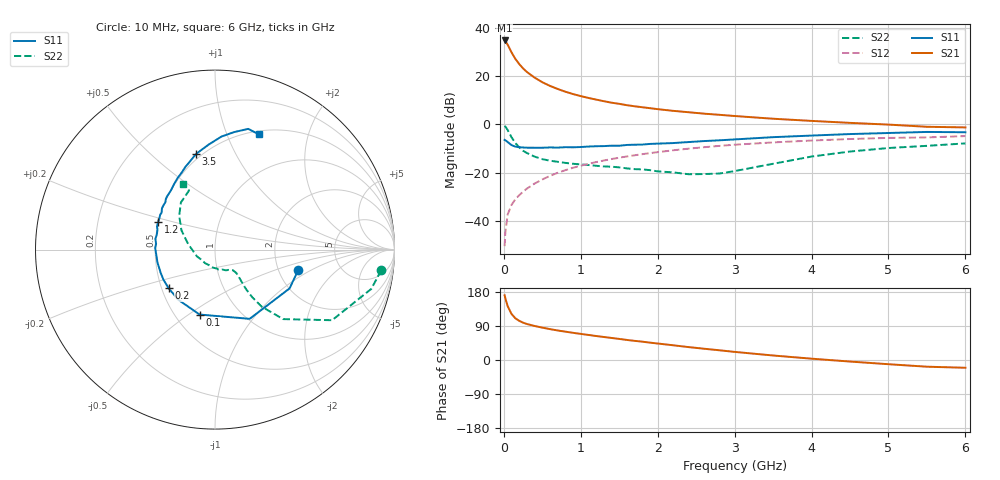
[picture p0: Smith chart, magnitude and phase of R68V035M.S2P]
! SIEMENS Small Signal Semiconductors
! BFR193
! Si NPN RF Bipolar Junction Transistor in SOT23
! VCE = 8 V  IC = 35 mA
! Common Emitter S-Parameters:  May  1996
# GHz  S  MA  R  50
!  f  S11  S21  S12  S22
! GHz  MAG  ANG  MAG  ANG  MAG  ANG  MAG  ANG
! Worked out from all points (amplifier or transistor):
!   36 points, 10 MHz to 6 GHz, reference 50 ohm
!   highest |S21| = 34.8 dB at 10 MHz (marker M1)
!   |S21| within 3 dB of that: start of sweep to 69.24 MHz
!   unconditionally stable (mu >= 1): 471.7 MHz to 2.129 GHz
!   at 250 MHz: K = 0.90, MSG = 25.5 dB, |S12| = -27.9 dB
!   at 1.4 GHz: K = 1.02, MAG = 10.8 dB, |S12| = -14.4 dB
!   at 6 GHz: K = 0.95, MSG = 1.8 dB, |S12| = -4.8 dB
!   S11 on the Smith chart (normalised r, x): 10 MHz: 2.56, -0.77; 100 MHz: 0.66, -0.55; 200 MHz: 0.54, -0.27; 1.2 GHz: 0.50, +0.18; 3.5 GHz: 0.47, +0.71; 6 GHz: 0.54, +1.30
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0.01  0.4773 -14.0  54.8 170.7  0.003 84.2  0.9328 -7.1
0.02  0.4684 -27.5  52.79 162.4  0.0059 77.1  0.8982 -14.1
0.05  0.4314 -63.4  44.61 142.0  0.0136 70.2  0.7617 -31.1
0.1  0.3719 -103.3  31.04 121.5  0.0215 66.5  0.5419 -45.6
0.15  0.3464 -126.2  22.76 110.0  0.0282 65.7  0.4107 -50.7
0.2  0.3362 -140.0  17.78 103.3  0.0341 67.6  0.3346 -52.0
0.25  0.3327 -149.3  14.45 98.5  0.0404 68.6  0.2846 -51.9
0.3  0.3291 -157.0  12.19 95.0  0.0467 70.0  0.2551 -51.2
0.4  0.3285 -167.4  9.298 89.8  0.0595 71.5  0.215 -49.6
0.5  0.3284 -175.0  7.469 85.4  0.0722 71.6  0.1904 -48.2
0.6  0.3332 178.7  6.271 81.5  0.0859 71.5  0.1769 -47.7
0.8  0.3374 169.7  4.754 74.8  0.1127 70.0  0.1594 -48.6
0.9  0.335 165.2  4.247 71.7  0.1265 69.0  0.1528 -48.9
1.1  0.3476 158.5  3.532 66.1  0.1523 67.1  0.144 -52.9
1.2  0.3529 153.7  3.263 63.3  0.1657 65.9  0.1388 -55.0
1.6  0.375 142.0  2.5 52.9  0.2166 60.4  0.1226 -67.0
2.2  0.4103 126.9  1.909 38.9  0.2906 52.0  0.1014 -95.7
2.8  0.4678 113.3  1.58 25.7  0.3583 43.0  0.0959 -145.4
3.5  0.5438 101.1  1.31 11.9  0.4232 32.2  0.1528 168.3
4.5  0.6304 86.8  1.075 -4.1  0.4974 18.3  0.2741 136.7
5.5  0.6977 74.6  0.892 -17.7  0.5372 4.5  0.3594 113.7
6  0.687 69.3  0.866 -20.5  0.5722 0.7  0.404 115.9
